(* Logix 5000 AddOnInstructionDefinition export QWX43; software revision 18.02 *)

TYPE SKT_Write_Parameters :
STRUCT
   Timeout : DINT;
   ToAddr : SKT_Address;
   Buffer : STR_480;
END_STRUCT
END_TYPE

TYPE SKT_Create_Parameters :
STRUCT
   Type : DINT;   // 1 - TCP 2- UPD
   Addr : SKT_Address;
END_STRUCT
END_TYPE

TYPE QWX43_Header :
STRUCT
   SOT : INT;   // Constant identifier that a transfer of new parameters starts. Always has the following value: 0xABCD.
   ProtocolVersion : INT;   // A version identifier of the protocol. Whenever a software version is released which has changes in the protocols (adding or removing parameters) the version is increased. The version starts with 1. Always 2
   SenderID : String40;   // PLC sends data to QWX43: OrderNr_SerialNr (null terminated string, 36 bytes long) Note: The sizes of the Sender ID is different when sending or receiving
   NrOfPar : INT;   // The total amount of transmitted parameters per transfer.
   NrOfBytes : INT;   // The total amount of bytes of all transmitted parameters.
END_STRUCT
END_TYPE

TYPE SKT_OpenConnection_Parameters :
STRUCT
   Timeout : DINT;
   DestAddr : STRING;
END_STRUCT
END_TYPE

TYPE SKT_Read_Parameters :
STRUCT
   Timeout : DINT;
   BufLen : DINT;
END_STRUCT
END_TYPE

TYPE SKT_Address :
STRUCT
   Family : INT;   // Address Family Must be 2
   Port : INT;   // Port Number
   Addr : SINT[4];   // IP Address
END_STRUCT
END_TYPE

TYPE QWX43_SensorData :
STRUCT
   temperature : REAL;   // °C
   speedOfSound : REAL;   // m/s
   viscosity : REAL;   // mPa/s
   concentrationCo2 : REAL;   // %mass
   TSOriginalGravity : REAL;   // %mass
   TSRealExtract : REAL;   // %mass
   originalGravity : REAL;   // °P
   realExtract : REAL;   // °P
   alcoholPercentMass : REAL;   // %mass
   alcoholPercentVolume : REAL;   // %vol
   densityAt20Degrees : REAL;   // g/cm³
   densityAt15Degrees : REAL;   // g/cm³
   realFermentationDegree : REAL;   // %
   fermentableSugars : REAL;   // %mass
   nonFermentableSugars : REAL;   // %mass
   apparentExtract : REAL;   // °P
   residualExtractBalling : REAL;   // °P
   alcoholBalling : REAL;   // %vol
   apparFermentationDeg : REAL;   // %
   fermentationSpeed : REAL;   // %vol/h
   viscosityAt20Degrees : REAL;   // mPa/s
   originalGravityMebak : REAL;   // °P
   realExtractMebak : REAL;   // °P
   alcoholPercentMassMebak : REAL;   // %mass
   alcoholPercentVolMebak : REAL;   // %vol
   densityAt20DegreesMebak : REAL;   // g/cm³
   densityAt15DegreesMebak : REAL;   // g/cm³
   realFermentationDegMebak : REAL;   // %
   apparentExtractMebak : REAL;   // °P
   residExtractBallingMebak : REAL;   // °P
   alcoholBallingMebak : REAL;   // %vol
   apparFermentationDegMebak : REAL;   // %
   errorCode : INT[10];   // -
   service_Temperature1 : REAL;   // °C
   service_Temperature2 : REAL;   // °C
   service_SSpeed : REAL;   // m/s
   service_SSpeedH2O : REAL;   // m/s
   service_dSSpeed : REAL;   // m/s
   service_Density45 : REAL;   // g/cm³
   service_Density : REAL;   // g/cm³
   service_DensityH2O : REAL;   // g/cm³
   service_RelDensity : REAL;   // g/cm³
   service_Viscosity : REAL;   // mPa/s
   service_TempElectronic : REAL;   // °C
   service_TOfRaw : REAL;   // s
   service_TransFrqc : REAL;   // Hz
   service_TDCError : INT;   // -
   service_DIVOFrqc : REAL;   // Hz
   service_DIVODamping : REAL;   // -
   service_DIVOCapacity : REAL;   // -
   service_DIVOStatus : REAL;   // -
   service_Uncovered : INT;   // -
END_STRUCT
END_TYPE

TYPE STR_480 :   // string type
STRUCT
   LEN : DINT;
   DATA : SINT[480];
END_STRUCT
END_TYPE

TYPE String40 :   // string type
STRUCT
   LEN : DINT;
   DATA : SINT[40];
END_STRUCT
END_TYPE

TYPE SKT_Read_Response :
STRUCT
   FromAddr : SKT_Address;
   Buffer : STR_480;
END_STRUCT
END_TYPE

TYPE SKT_DATA_CLIENT :
STRUCT
   Timeout : DINT;
   Create_Source : SKT_Create_Parameters;
   Instance : DINT;
   Connect_Source : SKT_OpenConnection_Parameters;
   Read_Source : SKT_Read_Parameters;
   Read_Response : SKT_Read_Response;
   Write_Source : SKT_Write_Parameters;
   Write_SizeSent : DINT;
END_STRUCT
END_TYPE

ADD_ON_INSTRUCTION SKT_AOI_TCP_CLIENT   (* revision 1.0, ExecutePrescan *)
VAR_IN_OUT
   Client_Data : SKT_DATA_CLIENT; {required}   // This tags holds all the data used by the messages
END_VAR
VAR_INPUT
   Enable_Socket : BOOL; {visible}   // Set by user to enable or disable socket
   Stop_On_Error : BOOL; {visible}   // If any message errors, then delete socket and stop
END_VAR
VAR_IN_OUT
   Create_MSG : MESSAGE; {required}   // Create socket
   Connect_MSG : MESSAGE; {required}   // Connect socket to server.
   Read_MSG : MESSAGE; {required}   // Message to tell socket to return any data it has recieved
   Write_MSG : MESSAGE; {required}   // Write socket message
   Delete_MSG : MESSAGE; {required}   // Delete socket
END_VAR
VAR_OUTPUT
   ENABLED : BOOL; {access Read Only, visible}   // Socket not currently open
   CONNECTING : BOOL; {access Read Only, visible}   // Trying to connect to Server.
   OPEN : BOOL; {access Read Only, visible}   // Socket connection Open
   READ : BOOL; {access Read Only, visible}   // New Data Ready - Set by AOI when a string is received, cleared by user to acknowledge
   WRITE : BOOL; {access Read Only, visible}   // Set this bit to Write Data
   ERROR : BOOL; {access Read Only, visible}   // A message had an Error
END_VAR
VAR
   State : DINT := 60;   // Current state
   lastport : DINT; {access None}
END_VAR

ROUTINE Logic   (* ladder *)
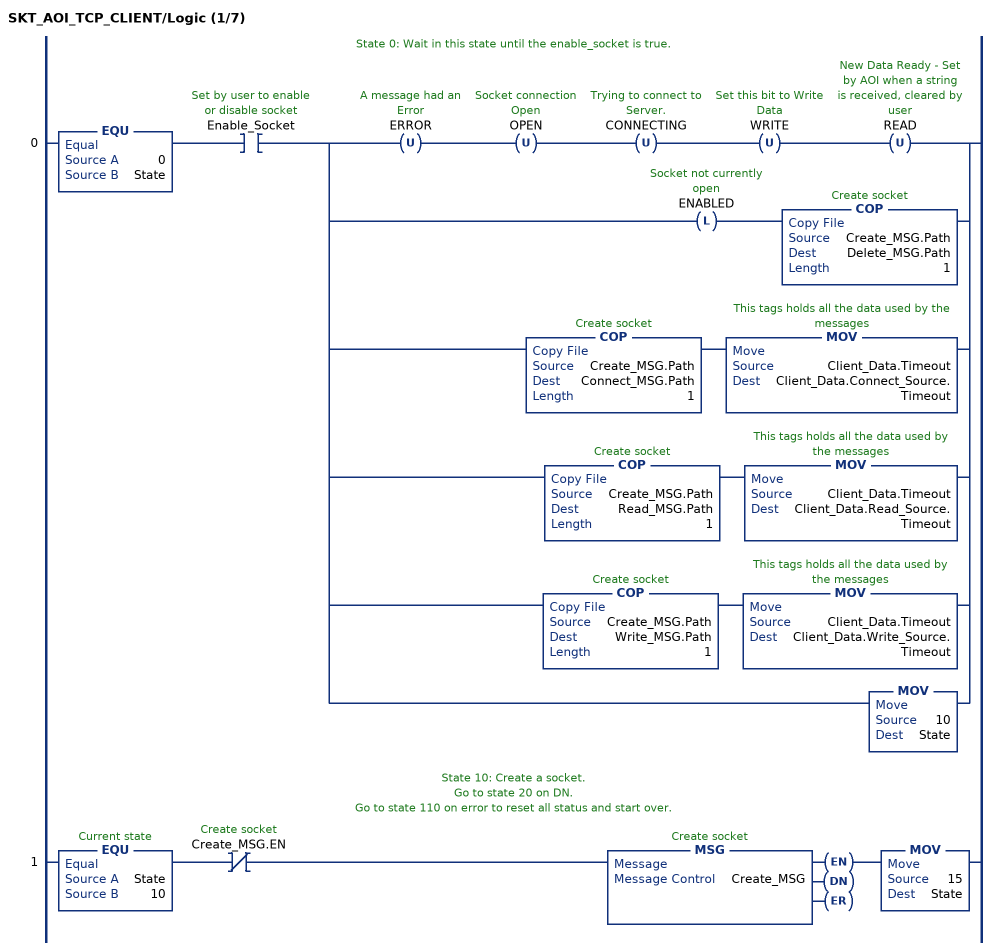
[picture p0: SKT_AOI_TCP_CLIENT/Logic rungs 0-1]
   // State 0: Wait in this state until the enable_socket is true.
   0: EQU(0,State)XIC(Enable_Socket)[OTU(ERROR) OTU(OPEN) OTU(CONNECTING) OTU(WRITE) OTU(READ) ,OTL(ENABLED) COP(Create_MSG.Path,Delete_MSG.Path,1) ,COP(Create_MSG.Path,Connect_MSG.Path,1) MOV(Client_Data.Timeout,Client_Data.Connect_Source.Timeout) ,COP(Create_MSG.Path,Read_MSG.Path,1) MOV(Client_Data.Timeout,Client_Data.Read_Source.Timeout) ,COP(Create_MSG.Path,Write_MSG.Path,1) MOV(Client_Data.Timeout,Client_Data.Write_Source.Timeout) ,MOV(10,State) ];
   // State 10: Create a socket.
   // Go to state 20 on DN.
   // Go to state 110 on error to reset all status and start over.
   1: EQU(State,10)XIO(Create_MSG.EN)MSG(Create_MSG)MOV(15,State);
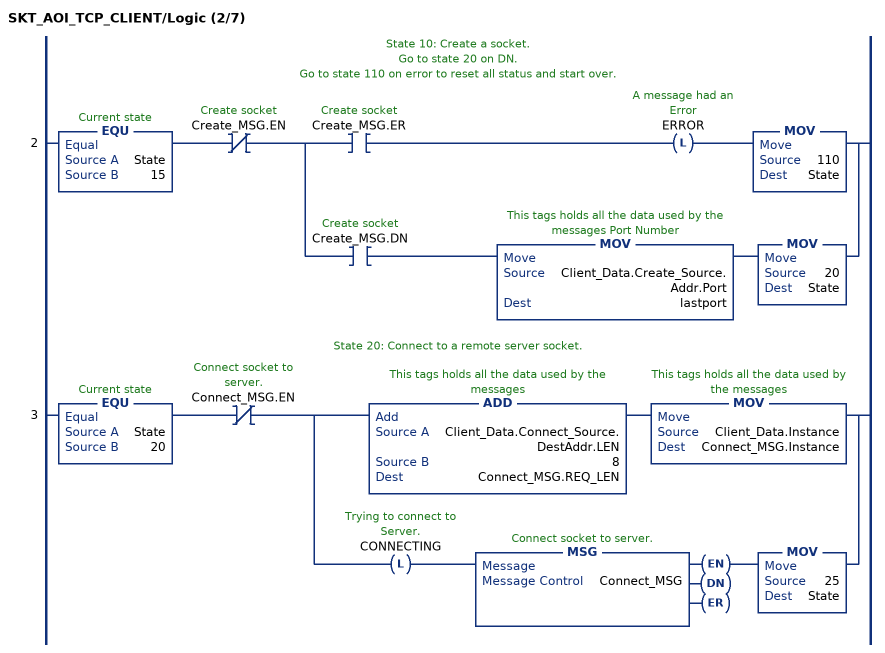
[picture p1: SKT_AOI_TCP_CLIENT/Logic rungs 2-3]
   // State 10: Create a socket.
   // Go to state 20 on DN.
   // Go to state 110 on error to reset all status and start over.
   2: EQU(State,15)XIO(Create_MSG.EN)[XIC(Create_MSG.ER) OTL(ERROR) MOV(110,State) ,XIC(Create_MSG.DN) MOV(Client_Data.Create_Source.Addr.Port,lastport) MOV(20,State) ];
   // State 20: Connect to a remote server socket.
   3: EQU(State,20)XIO(Connect_MSG.EN)[ADD(Client_Data.Connect_Source.DestAddr.LEN,8,Connect_MSG.REQ_LEN) MOV(Client_Data.Instance,Connect_MSG.Instance) ,OTL(CONNECTING) MSG(Connect_MSG) MOV(25,State) ];
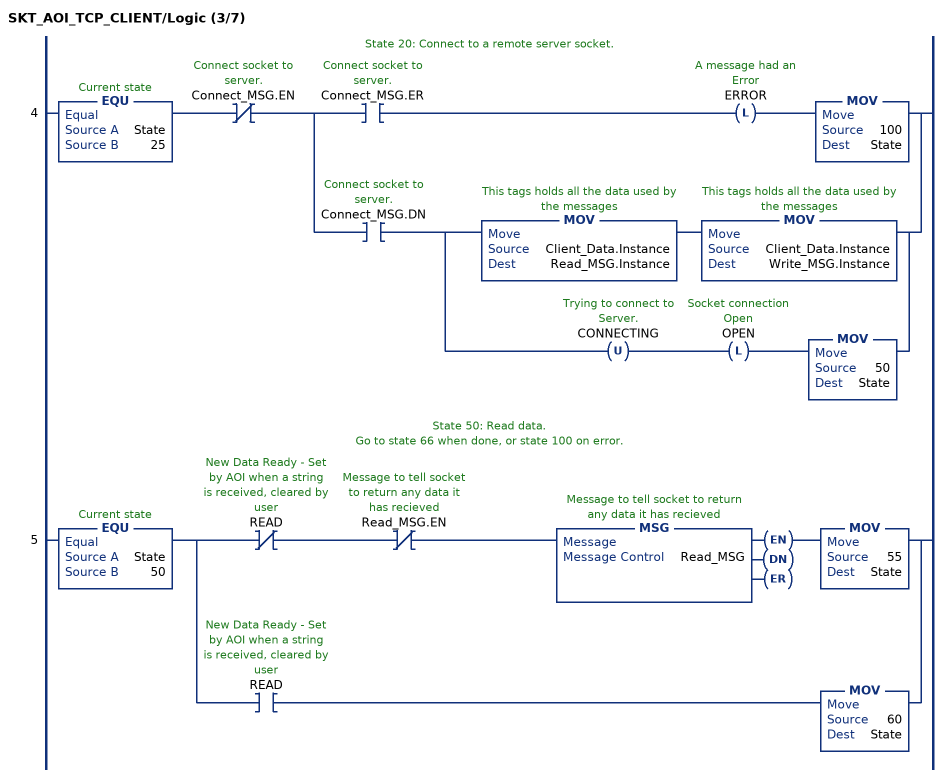
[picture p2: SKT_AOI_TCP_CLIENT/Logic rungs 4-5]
   // State 20: Connect to a remote server socket.
   4: EQU(State,25)XIO(Connect_MSG.EN)[XIC(Connect_MSG.ER) OTL(ERROR) MOV(100,State) ,XIC(Connect_MSG.DN) [MOV(Client_Data.Instance,Read_MSG.Instance) MOV(Client_Data.Instance,Write_MSG.Instance) ,OTU(CONNECTING) OTL(OPEN) MOV(50,State) ] ];
   // State 50: Read data.
   // Go to state 66 when done, or state 100 on error.
   5: EQU(State,50)[XIO(READ) XIO(Read_MSG.EN) MSG(Read_MSG) MOV(55,State) ,XIC(READ) MOV(60,State) ];
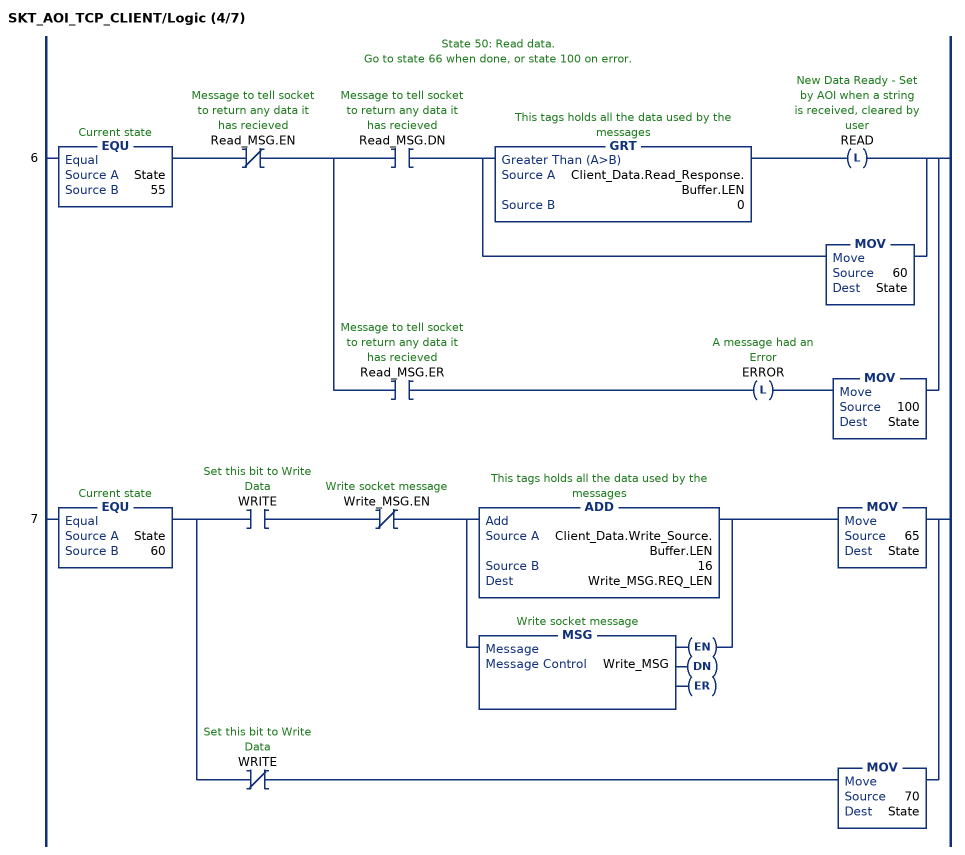
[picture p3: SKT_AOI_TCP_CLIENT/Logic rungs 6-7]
   // State 50: Read data.
   // Go to state 66 when done, or state 100 on error.
   6: EQU(State,55)XIO(Read_MSG.EN)[XIC(Read_MSG.DN) [GRT(Client_Data.Read_Response.Buffer.LEN,0) OTL(READ) ,MOV(60,State) ] ,XIC(Read_MSG.ER) OTL(ERROR) MOV(100,State) ];
   7: EQU(State,60)[XIC(WRITE) XIO(Write_MSG.EN) [ADD(Client_Data.Write_Source.Buffer.LEN,16,Write_MSG.REQ_LEN) ,MSG(Write_MSG) ] MOV(65,State) ,XIO(WRITE) MOV(70,State) ];
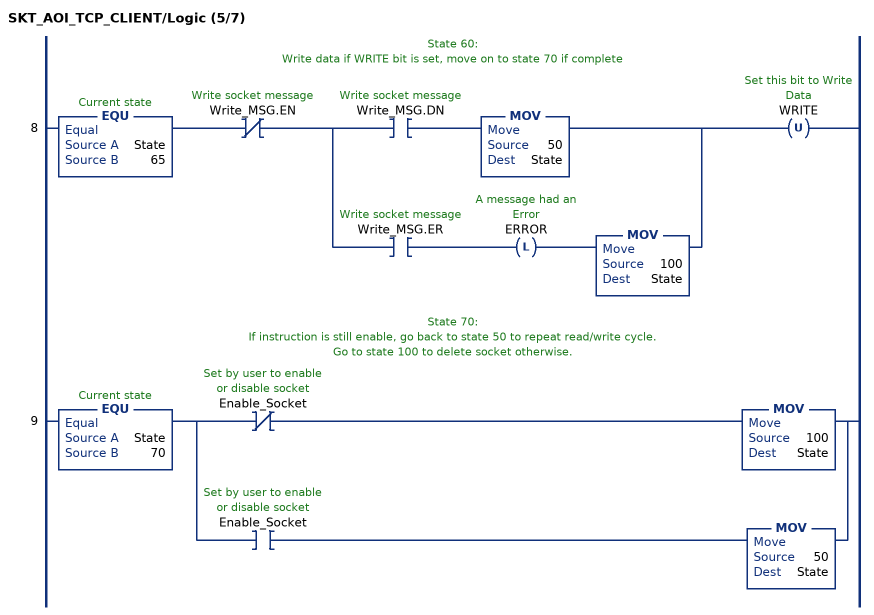
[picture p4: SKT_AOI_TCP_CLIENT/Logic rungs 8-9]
   // State 60:
   // Write data if WRITE bit is set, move on to state 70 if complete
   8: EQU(State,65)XIO(Write_MSG.EN)[XIC(Write_MSG.DN) MOV(50,State) ,XIC(Write_MSG.ER) OTL(ERROR) MOV(100,State) ]OTU(WRITE);
   // State 70:
   // If instruction is still enable, go back to state 50 to repeat read/write cycle.
   // Go to state 100 to delete socket otherwise.
   9: EQU(State,70)[XIO(Enable_Socket) MOV(100,State) ,XIC(Enable_Socket) MOV(50,State) ];
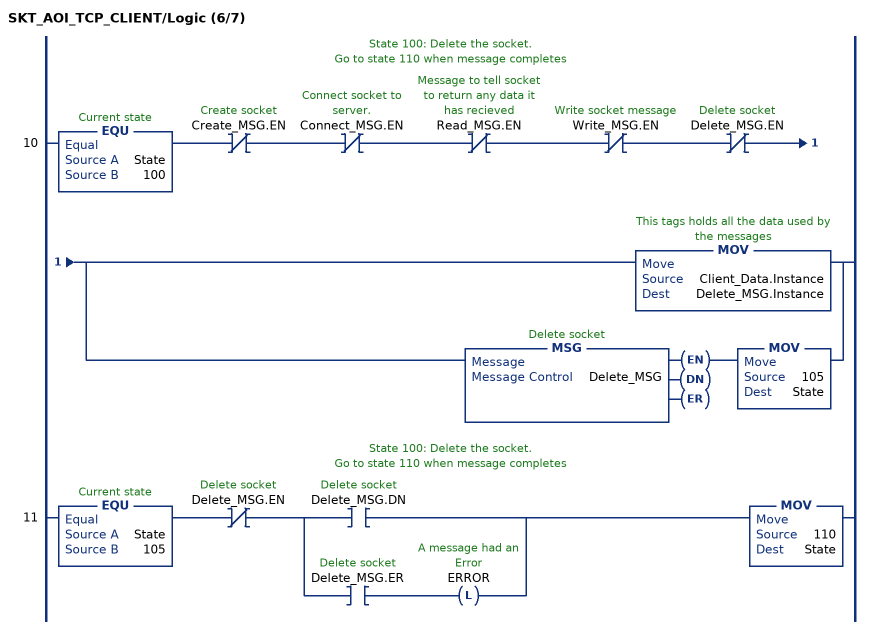
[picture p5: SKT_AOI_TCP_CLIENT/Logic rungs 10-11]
   // State 100: Delete the socket.
   // Go to state 110 when message completes
   10: EQU(State,100)XIO(Create_MSG.EN)XIO(Connect_MSG.EN)XIO(Read_MSG.EN)XIO(Write_MSG.EN)XIO(Delete_MSG.EN)[MOV(Client_Data.Instance,Delete_MSG.Instance) ,MSG(Delete_MSG) MOV(105,State) ];
   // State 100: Delete the socket.
   // Go to state 110 when message completes
   11: EQU(State,105)XIO(Delete_MSG.EN)[XIC(Delete_MSG.DN) ,XIC(Delete_MSG.ER) OTL(ERROR) ]MOV(110,State);
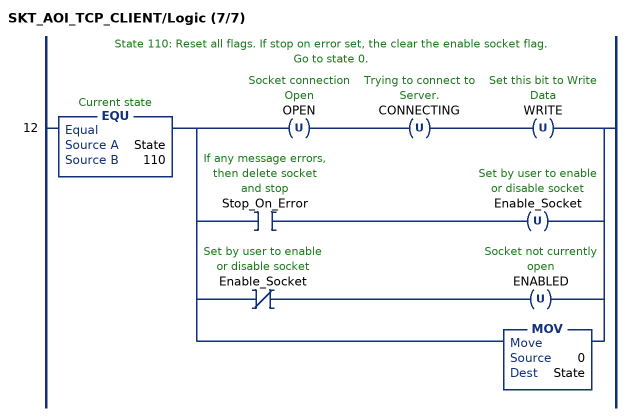
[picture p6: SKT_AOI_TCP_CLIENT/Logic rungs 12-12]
   // State 110: Reset all flags. If stop on error set, the clear the enable socket flag.
   // Go to state 0.
   12: EQU(State,110)[OTU(OPEN) OTU(CONNECTING) OTU(WRITE) ,XIC(Stop_On_Error) OTU(Enable_Socket) ,XIO(Enable_Socket) OTU(ENABLED) ,MOV(0,State) ];
END_ROUTINE

ROUTINE Prescan   (* ladder *)
// Prescan
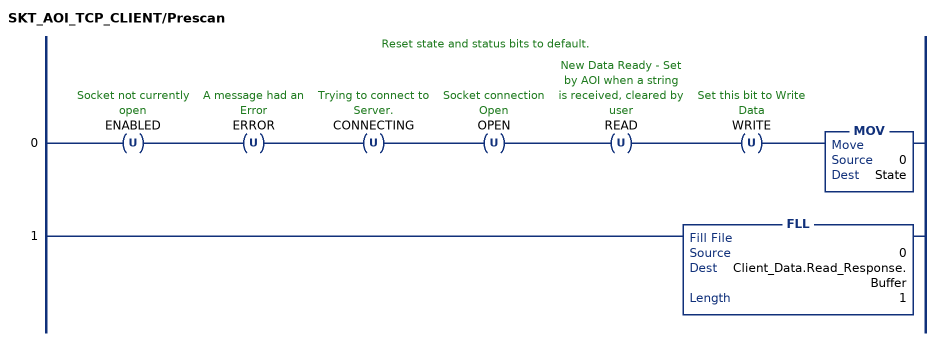
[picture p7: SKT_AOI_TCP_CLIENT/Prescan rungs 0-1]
   // Reset state and status bits to default.
   0: OTU(ENABLED)OTU(ERROR)OTU(CONNECTING)OTU(OPEN)OTU(READ)OTU(WRITE)MOV(0,State);
   1: FLL(0,Client_Data.Read_Response.Buffer,1);
END_ROUTINE
END_ADD_ON_INSTRUCTION

ADD_ON_INSTRUCTION QWX43   (* revision 1.1, vendor Endress+Hauser *)
// TCP/IP Communication to a QWX43 sensor
// Revision note:
// V1.01
// fixed that the Output Buffer was not copied to the send data
// Protocol Revision 3
// Help:
// Communication Handler for Endress+Hauser QWX43 Sensor.
// Communication is handled over TCP/IP. The Sensor will transmit and receive data on Port 50000.
// Protocol definition - Version 3
// Header [38 Bytes] - StartOfTransfer | Version | SenderID | NumberOfParameters | NrOfBytes
// Sensor Data [220 Bytes]
// Trailer [2 Bytes] - EndOfTransfer
// Revision:
// v1.0 - Initial release
// ***************************************************************************
// Message Paths
//     5570 and 5560 controllers
//         It will be 1,[Slot of ethernet module] if typed manually, or '$01$xx'if loaded programmatically to the .PATH field where xx is the HEX equivalent of decimal value of the slot. (ex. Slot 12 in HEX would be 0C)
//     5370 controllers
//         It will be 1,0 if typed manually, or '$01$00' if loaded programmatically to the .PATH field.
//     5380 controllers
//         Linear/ DLR mode
//             1,0 is the preferred recommended path to self, or '$01$00' if loaded programmatically the .PATH field.
//         Dual IP mode
//             If the controller is in dual IP mode the message path will be the same as above however the source of the CREATE MESSAGE needs to have the IP of the port that the socket will communicate
//             Reference QA48896 - 5380 Ethernet Socket Errors and Path Information  to specify the correct port the message should sent out for dual IP
// Note: 'THIS' will not work as the path for the 5380 controllers because of the dual IP capabilities use the path provided above
//     5580 controllers
//         When doing a message to self the message path should either be '1,<slot of controller>' or THIS. THIS is the preferred recommended path to self, or '$1F$00$00$00';if loaded programmatically the .PATH field.
// see also: IN37624 Socket Communication in ControlLogix, CompactLogix and MicroLogix Controllers
// https://rockwellautomation.custhelp.com/app/answers/answer_view/a_id/470690
// ***************************************************************************
// The DestAddr holds the IP and port adress of the QWX43 in the Format "192.168.1.127?port=50000"
VAR_INPUT
   Inp_Release : BOOL; {visible}   // 1= Enable communication to QWX43
   Inp_MaxPressure : REAL; {visible}   // Maximum head pressure of the tank in bar (absolute pressure)
END_VAR
VAR_IN_OUT
   SKT_DATA_Client : SKT_DATA_CLIENT; {required}   // This tags holds all the data used by the messages
   SKT_MSG_Client_Create : MESSAGE; {required}   // Create socket
   SKT_MSG_Client_Connect : MESSAGE; {required}   // Connect socket to server.
   SKT_MSG_Client_Read : MESSAGE; {required}   // Message to tell socket to return any data it has recieved
   SKT_MSG_Client_Write : MESSAGE; {required}   // Write socket message
   SKT_MSG_Client_Delete : MESSAGE; {required}   // Delete socket
   SKT_MSG_Delete_All : MESSAGE; {required}   // Delete all sockets in modul
   Out_SensorData : QWX43_SensorData; {required}   // Received Sensor Data
END_VAR
VAR_INPUT
   Cfg_ComModuleSingleUse : BOOL; {visible}   // The configured communication module is 1=only used for this QWX43 0=also used by others (default)
END_VAR
VAR_OUTPUT
   Sts_Error : BOOL; {access Read Only, visible}   // 1= functionblock is in an error state
   Sts_State : DINT; {access Read Only, visible}   // State of the function 0=Wait, 1=Connect, 2=Send, 3=Receive 100=ConfigError, 101=ConnectionError, 102=TelegramError, 103=VersionError
END_VAR
VAR
   Err_Config : BOOL; {access None}   // Error in basic configuration
   Wrk_State : DINT; {access None}   // State of the function 0=Wait, 1=Connect, 2=Send, 3=Receive 100=ConfigError, 101=ConnectionError, 102=TelegramError, 103=VersionError
   ons : DINT; {access None}
   Wrk_Connected : BOOL; {access None}   // Socket is connected to the QWX43
   SKT_AOI_Client : SKT_AOI_TCP_CLIENT;   // Socket handling
   Wrk_SendInterval_T : TIMER := (PRE := 1000); {access None}
   cSOT : INT := 16#abcd; {access None}   // 0xABCD
   cEOT : INT := 16#fedc; {access None}   // 0xFEDC
   Wrk_SendHeader : QWX43_Header := (SOT := 16#abcd, ProtocolVersion := 3, SenderID := 'CLX', NrOfPar := 2, NrOfBytes := 6); {access None}
   Wrk_ReceiveHeader : QWX43_Header; {access None}
   Wrk_SendBytes : DINT := 56; {access None}
   Cfg_BytesHeader : DINT := 48; {access None}   // Number of bytes in header
   Cfg_BytesTrailer : DINT := 2; {access None}   // Number of bytes in trailer
   Cfg_BytesSendData : DINT := 6; {access None}   // Number of bytes in send data
   Wrk_SendBuffer : STR_480; {access None}
   Wrk_SendByteOffset : DINT; {access None}
   Wrk_SendByteLen : DINT; {access None}
   Wrk_dummyINT : INT; {access None}
   Wrk_ErrorCodePLC : INT; {access None}   // 0=no error (not used at the moment)
   Wrk_dummyDINT : DINT; {access None}
   Wrk_ReceiveBuffer : STR_480; {access None}
   Err_ReceiveDataLenNOK : BOOL; {access None}   // The received data lengh did not match
   Err_ReceiveHeaderDataNOK : BOOL; {access None}   // At least one of the received header data was incorrect
   Wrk_ReceiveBytesExpected : DINT := 270; {access None}   // Expected number of bytes to receive
   Cfg_BytesReceiveData : DINT := 220; {access None}   // Number of bytes in receive data
   Wrk_ReceiveByteOffset : DINT; {access None}
   Wrk_ReceiveByteLen : DINT; {access None}
   Wrk_ReceiveByteOffsetEOT : DINT; {access None}
   Wrk_ReceiveEOT : INT; {access None}
   Wrk_ReceiveSwapIndex : DINT; {access None}
   Wrk_ReceiveSwapNo : DINT; {access None}   // Number of data elements to swap
   Wrk_ReceiveSwapSize : DINT; {access None}   // Number of bytes per element to swap
   Wrk_dummyDINT_A : DINT[100]; {access None}
   Wrk_dummyINT_A : INT[100]; {access None}
   Wrk_dummyDINT_A_Size : DINT; {access None}
   Wrk_dummyINT_A_Size : DINT; {access None}
   Wrk_ReceiveBuffer_Size : DINT := 480; {access None}
   Wrk_SendBuffer_Size : DINT := 480; {access None}
   Err_ReceiveVersionNOK : BOOL; {access None}   // The received data version is incorrect
   Err_Connection : BOOL; {access None}   // No connection could be established
   Wrk_ConnectingError_T : TIMER := (PRE := 5000); {access None}
   Err_ConnectionTimeout : BOOL; {access None}   // Timeout after a connection was established
   Wrk_ConnectionTimeout_T : TIMER := (PRE := 5000); {access None}
   Wrk_CloseSocket : BOOL; {access None}   // Temporary close socket after a timeout
   Wrk_ConnectionTimeoutWait_T : TIMER := (PRE := 15000); {access None}
   Cfg_ConnectionTimeout : DINT := 5000; {access None}   // Timeout after a connection was opened, no data received [ms]
   Cfg_ConnectionTimeoutWait : DINT := 15000; {access None}   // Wait after a timeout befor trying to reconnect [ms]
   Cfg_ConnectionError : DINT := 5000; {access None}   // A connection could not be established [ms]
   Cfg_SendInterval : DINT := 1000; {access None}   // Intervaltime [ms]
   Err_MSGDeleteAll : BOOL; {access None}   // The MSG Delete All had an error
END_VAR

ROUTINE Logic   (* ladder *)
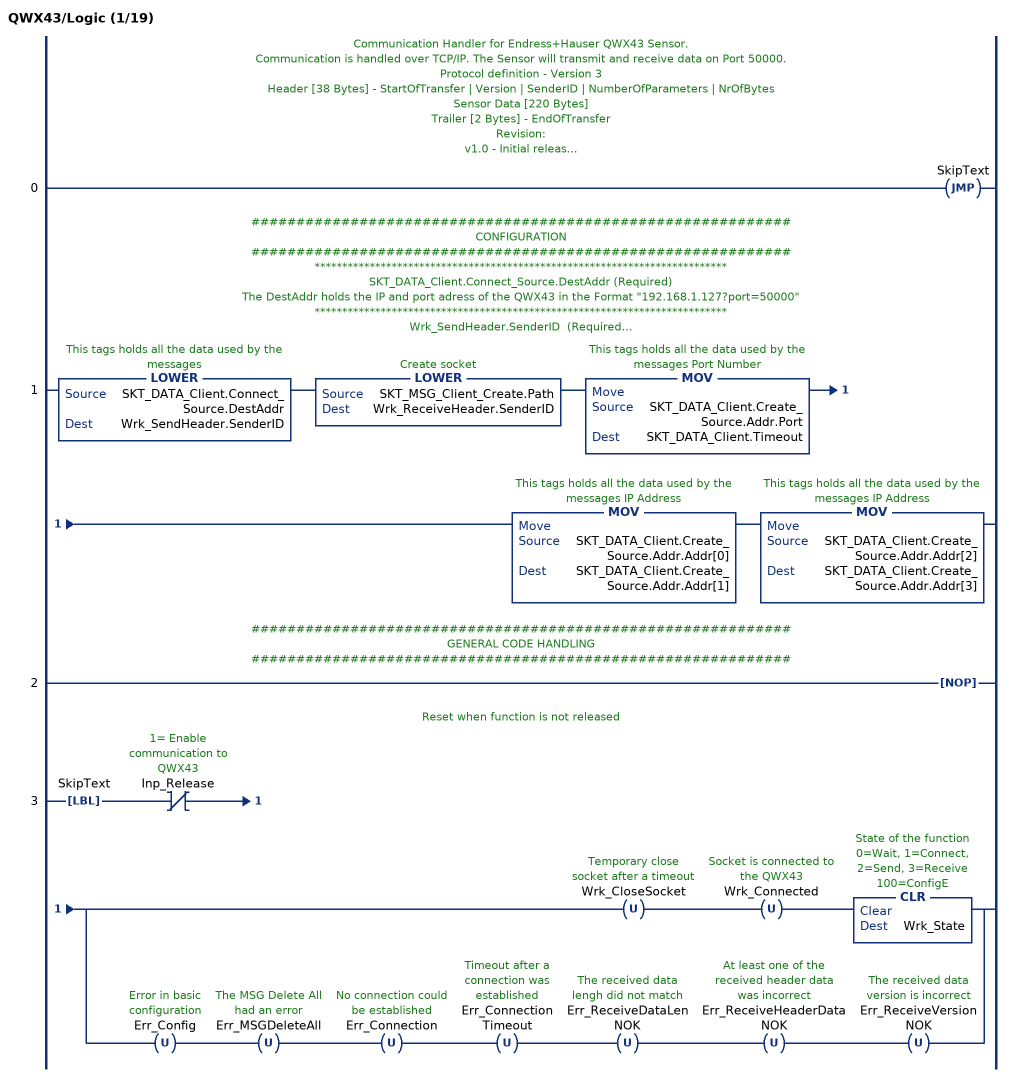
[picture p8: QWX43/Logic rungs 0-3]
   // Communication Handler for Endress+Hauser QWX43 Sensor.
   // Communication is handled over TCP/IP. The Sensor will transmit and receive data on Port 50000.
   // Protocol definition - Version 3
   // Header [38 Bytes] - StartOfTransfer | Version | SenderID | NumberOfParameters | NrOfBytes
   // Sensor Data [220 Bytes]
   // Trailer [2 Bytes] - EndOfTransfer
   // Revision:
   // v1.0 - Initial release
   // ***************************************************************************
   // In order to make it easier to find and configure these STRINGs, this rung
   // was added.  THE JMP (and the LBL on the following rung)
   // MUST NOT BE REMOVED!!!
   0: JMP(SkipText);
   // ############################################################
   // CONFIGURATION
   // ############################################################
   // ***************************************************************************
   // SKT_DATA_Client.Connect_Source.DestAddr (Required)
   // The DestAddr holds the IP and port adress of the QWX43 in the Format "192.168.1.127?port=50000"
   // ***************************************************************************
   // Wrk_SendHeader.SenderID  (Required)
   // This is a String which holds the Sender ID of the PLC (max 36 characters)
   // ***************************************************************************
   // SKT_MSG_Client_Create.Path  (Required, either here manualy or at the MSG instance at the AOI)
   // Message Paths
   //     5570 and 5560 controllers
   //         It will be 1,[Slot of ethernet module] if typed manually, or '$01$xx'if loaded programmatically to the .PATH field where xx is the HEX equivalent of decimal value of the slot. (ex. Slot 12 in HEX would be 0C)
   //     5370 controllers
   //         It will be 1,0 if typed manually, or '$01$00' if loaded programmatically to the .PATH field.
   //     5380 controllers
   //         Linear/ DLR mode
   //             1,0 is the preferred recommended path to self, or '$01$00' if loaded programmatically the .PATH field.
   //         Dual IP mode
   //             If the controller is in dual IP mode the message path will be the same as above however the source of the CREATE MESSAGE needs to have the IP of the port that the socket will communicate
   //             Reference QA48896 - 5380 Ethernet Socket Errors and Path Information  to specify the correct port the message should sent out for dual IP
   // Note: 'THIS' will not work as the path for the 5380 controllers because of the dual IP capabilities use the path provided above
   //     5580 controllers
   //         When doing a message to self the message path should either be '1,<slot of controller>' or THIS. THIS is the preferred recommended path to self, or '$1F$00$00$00';if loaded programmatically the .PATH field.
   // see also: IN37624 Socket Communication in ControlLogix, CompactLogix and MicroLogix Controllers
   // https://rockwellautomation.custhelp.com/app/answers/answer_view/a_id/470690
   // ***************************************************************************
   // Wrk_ReceiveHeader.SenderID (Only to visualize)
   // The Sender ID received from the QWX43
   // ***************************************************************************
   // SKT_DATA_Client.Create_Source.Addr.Port (Otpional)
   // Specify the local port number on which an application listens and receives. (Values 1 - 32767)
   // If you want a port that is randomly assigned, use port 0 (Default).
   // ***************************************************************************
   // SKT_DATA_Client.Timeout (Optional)
   // Defines how long the read instruction will wait for new data and block a write command
   // slower values is better for response time after a write command but increases the burden on th ecommunication module
   // the default value of 100ms should fit in most cases.
   // ***************************************************************************
   // SKT_DATA_Client.Create_Source.Addr.Addr[0] - [3] (Required for Dual IP)
   // When dual IP is used (for example with Compact Logix CPUs) then the IP address of the used Port must be configured.
   // Addr[0] holds the first (lowest) octet and Addr[3] thie last (highest) octet in HEX
   // for example: 192.168.1.11 would be:
   // Addr[0] = 16#0b (11)
   // Addr[1] = 16#01 (1)
   // Addr[2] = 16#a8 (168)
   // Addr[3] = 16#c0 (192)
   // If this function is not used then all four values have to be 0 !!!
   1: LOWER(SKT_DATA_Client.Connect_Source.DestAddr,Wrk_SendHeader.SenderID)LOWER(SKT_MSG_Client_Create.Path,Wrk_ReceiveHeader.SenderID)MOV(SKT_DATA_Client.Create_Source.Addr.Port,SKT_DATA_Client.Timeout)MOV(SKT_DATA_Client.Create_Source.Addr.Addr[0],SKT_DATA_Client.Create_Source.Addr.Addr[1])MOV(SKT_DATA_Client.Create_Source.Addr.Addr[2],SKT_DATA_Client.Create_Source.Addr.Addr[3]);
   // ############################################################
   // GENERAL CODE HANDLING
   // ############################################################
   2: NOP();
   // Reset when function is not released
   3: LBL(SkipText)XIO(Inp_Release)[OTU(Wrk_CloseSocket) OTU(Wrk_Connected) CLR(Wrk_State) ,OTU(Err_Config) OTU(Err_MSGDeleteAll) OTU(Err_Connection) OTU(Err_ConnectionTimeout) OTU(Err_ReceiveDataLenNOK) OTU(Err_ReceiveHeaderDataNOK) OTU(Err_ReceiveVersionNOK) ];
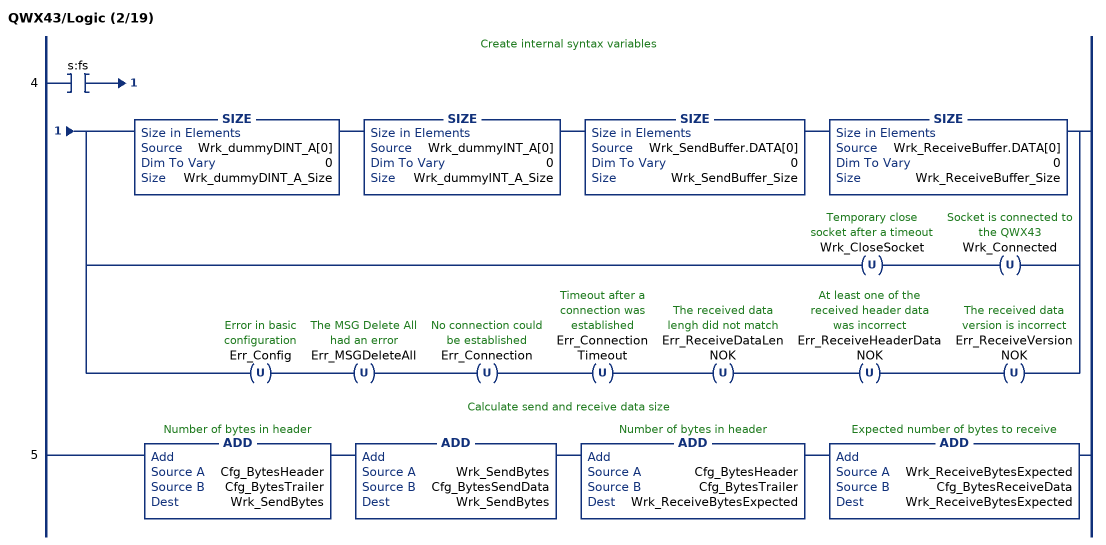
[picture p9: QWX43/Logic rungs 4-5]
   // Create internal syntax variables
   4: XIC(s:fs)[SIZE(Wrk_dummyDINT_A[0],0,Wrk_dummyDINT_A_Size) SIZE(Wrk_dummyINT_A[0],0,Wrk_dummyINT_A_Size) SIZE(Wrk_SendBuffer.DATA[0],0,Wrk_SendBuffer_Size) SIZE(Wrk_ReceiveBuffer.DATA[0],0,Wrk_ReceiveBuffer_Size) ,OTU(Wrk_CloseSocket) OTU(Wrk_Connected) ,OTU(Err_Config) OTU(Err_MSGDeleteAll) OTU(Err_Connection) OTU(Err_ConnectionTimeout) OTU(Err_ReceiveDataLenNOK) OTU(Err_ReceiveHeaderDataNOK) OTU(Err_ReceiveVersionNOK) ];
   // Calculate send and receive data size
   5: ADD(Cfg_BytesHeader,Cfg_BytesTrailer,Wrk_SendBytes)ADD(Wrk_SendBytes,Cfg_BytesSendData,Wrk_SendBytes)ADD(Cfg_BytesHeader,Cfg_BytesTrailer,Wrk_ReceiveBytesExpected)ADD(Wrk_ReceiveBytesExpected,Cfg_BytesReceiveData,Wrk_ReceiveBytesExpected);
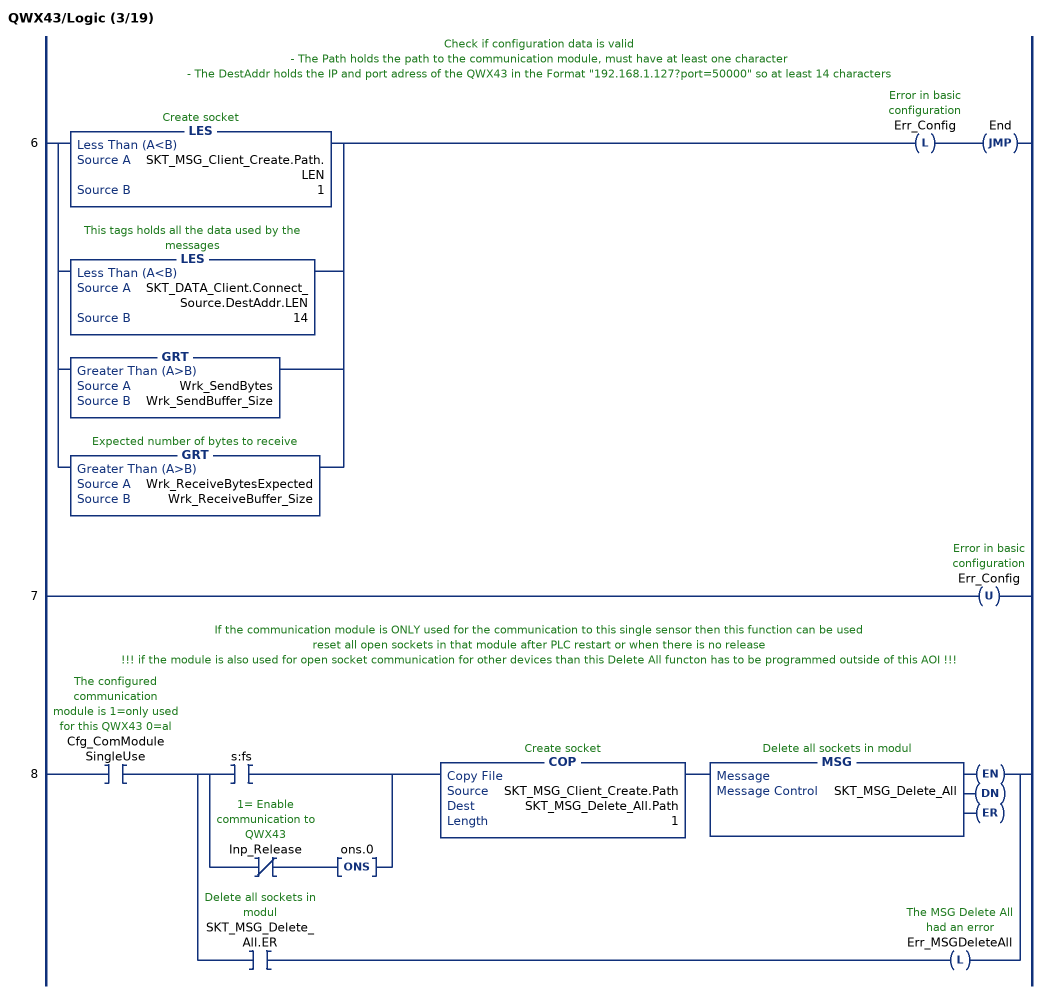
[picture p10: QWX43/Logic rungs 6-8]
   // Check if configuration data is valid
   // - The Path holds the path to the communication module, must have at least one character
   // - The DestAddr holds the IP and port adress of the QWX43 in the Format "192.168.1.127?port=50000" so at least 14 characters
   6: [LES(SKT_MSG_Client_Create.Path.LEN,1) ,LES(SKT_DATA_Client.Connect_Source.DestAddr.LEN,14) ,GRT(Wrk_SendBytes,Wrk_SendBuffer_Size) ,GRT(Wrk_ReceiveBytesExpected,Wrk_ReceiveBuffer_Size) ]OTL(Err_Config)JMP(End);
   7: OTU(Err_Config);
   // If the communication module is ONLY used for the communication to this single sensor then this function can be used
   // reset all open sockets in that module after PLC restart or when there is no release
   // !!! if the module is also used for open socket communication for other devices than this Delete All functon has to be programmed outside of this AOI !!!
   8: XIC(Cfg_ComModuleSingleUse)[[XIC(s:fs) ,XIO(Inp_Release) ONS(ons.0) ] COP(SKT_MSG_Client_Create.Path,SKT_MSG_Delete_All.Path,1) MSG(SKT_MSG_Delete_All) ,XIC(SKT_MSG_Delete_All.ER) OTL(Err_MSGDeleteAll) ];
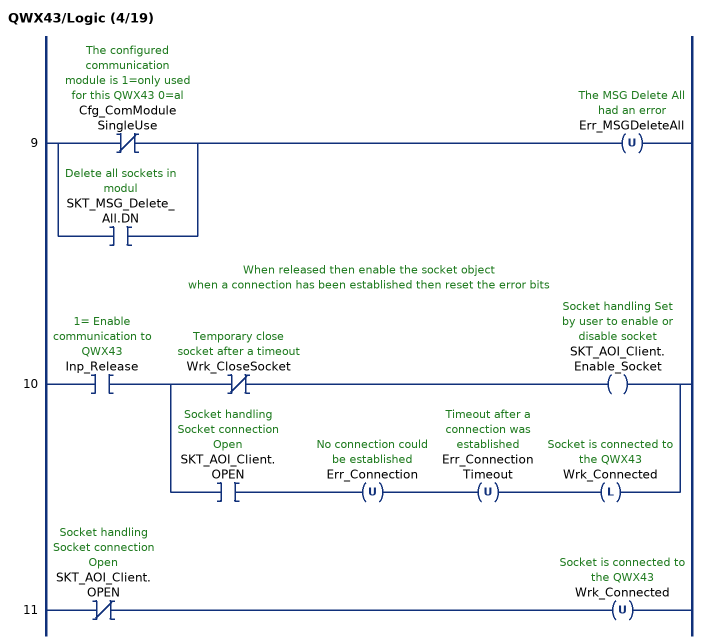
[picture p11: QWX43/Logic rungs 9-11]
   9: [XIO(Cfg_ComModuleSingleUse) ,XIC(SKT_MSG_Delete_All.DN) ]OTU(Err_MSGDeleteAll);
   // When released then enable the socket object
   // when a connection has been established then reset the error bits
   10: XIC(Inp_Release)[XIO(Wrk_CloseSocket) OTE(SKT_AOI_Client.Enable_Socket) ,XIC(SKT_AOI_Client.OPEN) OTU(Err_Connection) OTU(Err_ConnectionTimeout) OTL(Wrk_Connected) ];
   11: XIO(SKT_AOI_Client.OPEN)OTU(Wrk_Connected);
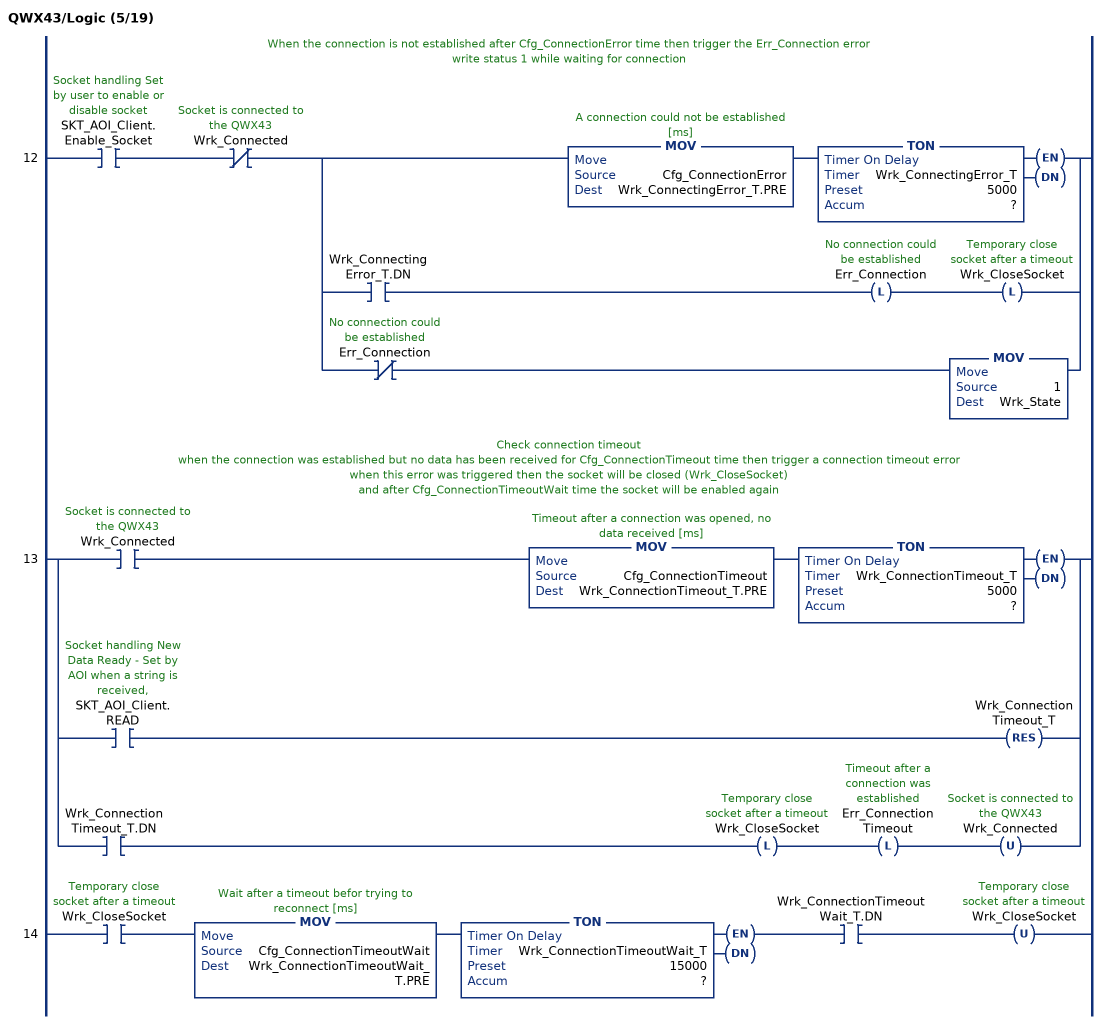
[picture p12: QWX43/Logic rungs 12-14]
   // When the connection is not established after Cfg_ConnectionError time then trigger the Err_Connection error
   // write status 1 while waiting for connection
   12: XIC(SKT_AOI_Client.Enable_Socket)XIO(Wrk_Connected)[MOV(Cfg_ConnectionError,Wrk_ConnectingError_T.PRE) TON(Wrk_ConnectingError_T,?,?) ,XIC(Wrk_ConnectingError_T.DN) OTL(Err_Connection) OTL(Wrk_CloseSocket) ,XIO(Err_Connection) MOV(1,Wrk_State) ];
   // Check connection timeout
   // when the connection was established but no data has been received for Cfg_ConnectionTimeout time then trigger a connection timeout error
   // when this error was triggered then the socket will be closed (Wrk_CloseSocket)
   // and after Cfg_ConnectionTimeoutWait time the socket will be enabled again
   13: [XIC(Wrk_Connected) MOV(Cfg_ConnectionTimeout,Wrk_ConnectionTimeout_T.PRE) TON(Wrk_ConnectionTimeout_T,?,?) ,XIC(SKT_AOI_Client.READ) RES(Wrk_ConnectionTimeout_T) ,XIC(Wrk_ConnectionTimeout_T.DN) OTL(Wrk_CloseSocket) OTL(Err_ConnectionTimeout) OTU(Wrk_Connected) ];
   14: XIC(Wrk_CloseSocket)MOV(Cfg_ConnectionTimeoutWait,Wrk_ConnectionTimeoutWait_T.PRE)TON(Wrk_ConnectionTimeoutWait_T,?,?)XIC(Wrk_ConnectionTimeoutWait_T.DN)OTU(Wrk_CloseSocket);
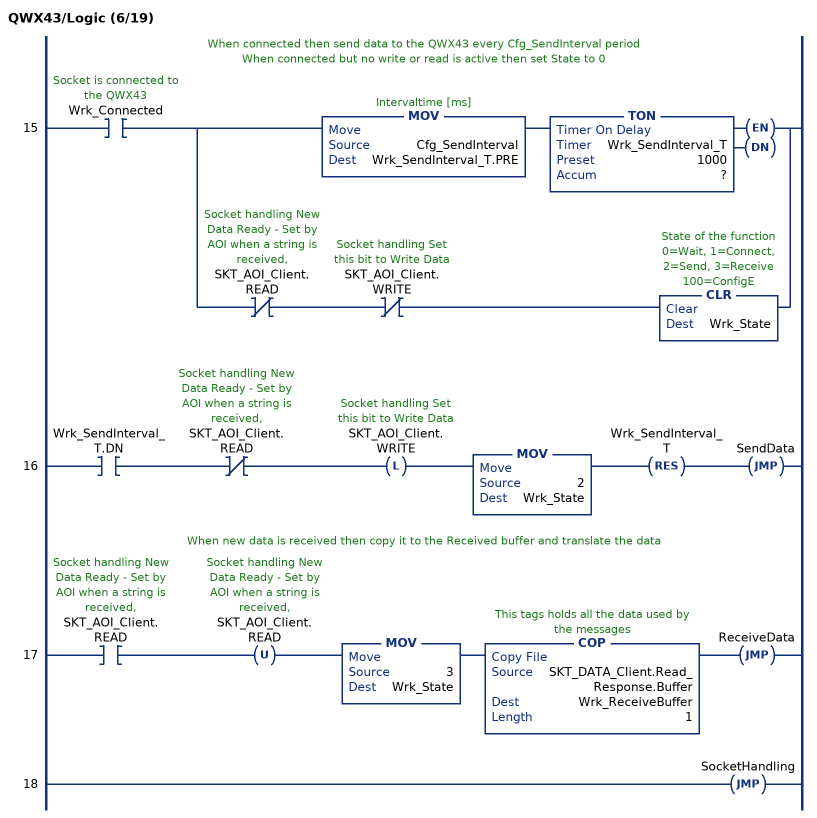
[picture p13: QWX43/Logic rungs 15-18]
   // When connected then send data to the QWX43 every Cfg_SendInterval period
   // When connected but no write or read is active then set State to 0
   15: XIC(Wrk_Connected)[MOV(Cfg_SendInterval,Wrk_SendInterval_T.PRE) TON(Wrk_SendInterval_T,?,?) ,XIO(SKT_AOI_Client.READ) XIO(SKT_AOI_Client.WRITE) CLR(Wrk_State) ];
   16: XIC(Wrk_SendInterval_T.DN)XIO(SKT_AOI_Client.READ)OTL(SKT_AOI_Client.WRITE)MOV(2,Wrk_State)RES(Wrk_SendInterval_T)JMP(SendData);
   // When new data is received then copy it to the Received buffer and translate the data
   17: XIC(SKT_AOI_Client.READ)OTU(SKT_AOI_Client.READ)MOV(3,Wrk_State)COP(SKT_DATA_Client.Read_Response.Buffer,Wrk_ReceiveBuffer,1)JMP(ReceiveData);
   18: JMP(SocketHandling);
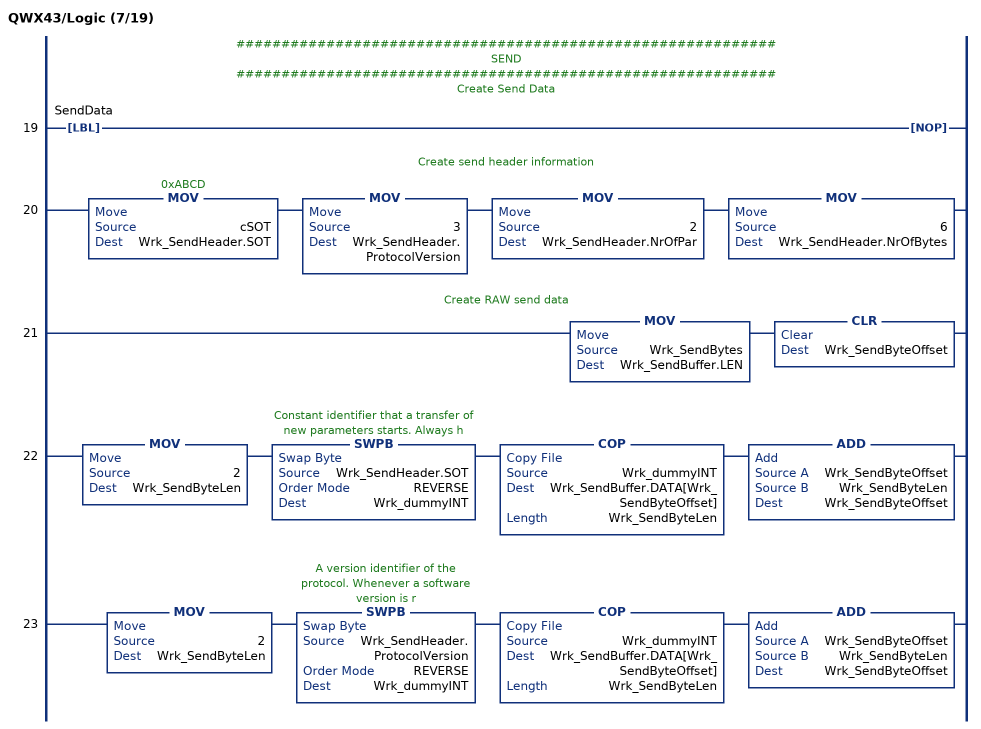
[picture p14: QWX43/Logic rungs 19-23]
   // ############################################################
   // SEND
   // ############################################################
   // Create Send Data
   19: LBL(SendData)NOP();
   // Create send header information
   20: MOV(cSOT,Wrk_SendHeader.SOT)MOV(3,Wrk_SendHeader.ProtocolVersion)MOV(2,Wrk_SendHeader.NrOfPar)MOV(6,Wrk_SendHeader.NrOfBytes);
   // Create RAW send data
   21: MOV(Wrk_SendBytes,Wrk_SendBuffer.LEN)CLR(Wrk_SendByteOffset);
   22: MOV(2,Wrk_SendByteLen)SWPB(Wrk_SendHeader.SOT,REVERSE,Wrk_dummyINT)COP(Wrk_dummyINT,Wrk_SendBuffer.DATA[Wrk_SendByteOffset],Wrk_SendByteLen)ADD(Wrk_SendByteOffset,Wrk_SendByteLen,Wrk_SendByteOffset);
   23: MOV(2,Wrk_SendByteLen)SWPB(Wrk_SendHeader.ProtocolVersion,REVERSE,Wrk_dummyINT)COP(Wrk_dummyINT,Wrk_SendBuffer.DATA[Wrk_SendByteOffset],Wrk_SendByteLen)ADD(Wrk_SendByteOffset,Wrk_SendByteLen,Wrk_SendByteOffset);
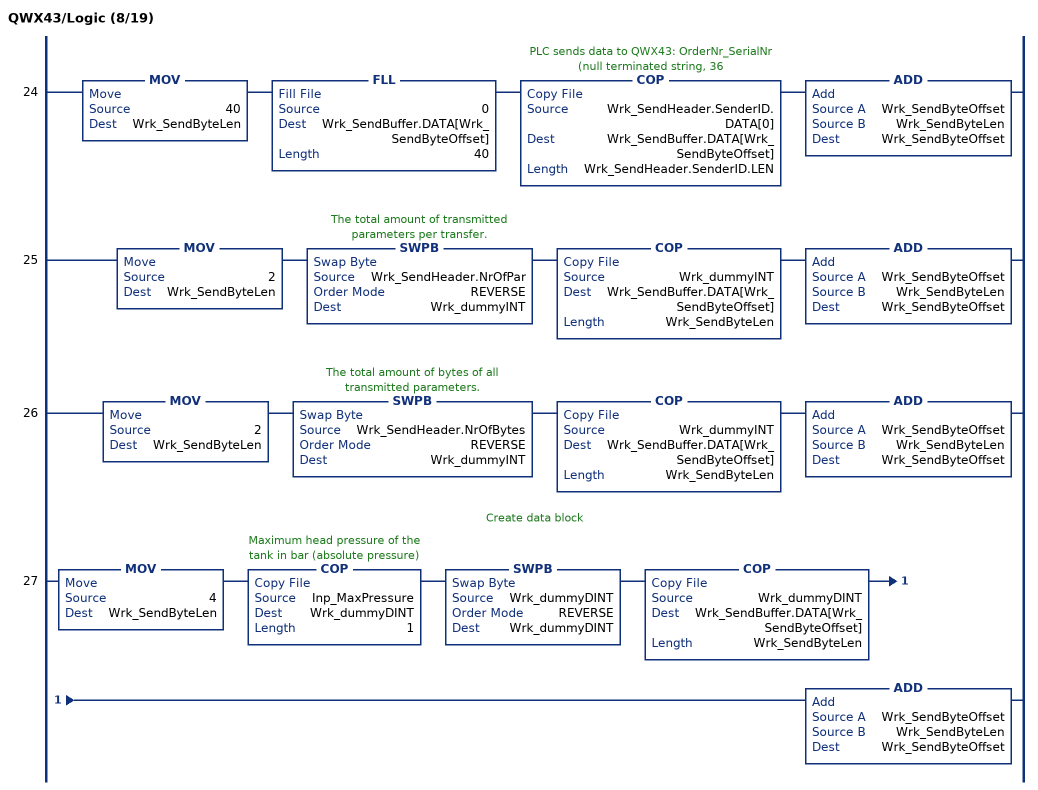
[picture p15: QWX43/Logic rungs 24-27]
   24: MOV(40,Wrk_SendByteLen)FLL(0,Wrk_SendBuffer.DATA[Wrk_SendByteOffset],40)COP(Wrk_SendHeader.SenderID.DATA[0],Wrk_SendBuffer.DATA[Wrk_SendByteOffset],Wrk_SendHeader.SenderID.LEN)ADD(Wrk_SendByteOffset,Wrk_SendByteLen,Wrk_SendByteOffset);
   25: MOV(2,Wrk_SendByteLen)SWPB(Wrk_SendHeader.NrOfPar,REVERSE,Wrk_dummyINT)COP(Wrk_dummyINT,Wrk_SendBuffer.DATA[Wrk_SendByteOffset],Wrk_SendByteLen)ADD(Wrk_SendByteOffset,Wrk_SendByteLen,Wrk_SendByteOffset);
   26: MOV(2,Wrk_SendByteLen)SWPB(Wrk_SendHeader.NrOfBytes,REVERSE,Wrk_dummyINT)COP(Wrk_dummyINT,Wrk_SendBuffer.DATA[Wrk_SendByteOffset],Wrk_SendByteLen)ADD(Wrk_SendByteOffset,Wrk_SendByteLen,Wrk_SendByteOffset);
   // Create data block
   27: MOV(4,Wrk_SendByteLen)COP(Inp_MaxPressure,Wrk_dummyDINT,1)SWPB(Wrk_dummyDINT,REVERSE,Wrk_dummyDINT)COP(Wrk_dummyDINT,Wrk_SendBuffer.DATA[Wrk_SendByteOffset],Wrk_SendByteLen)ADD(Wrk_SendByteOffset,Wrk_SendByteLen,Wrk_SendByteOffset);
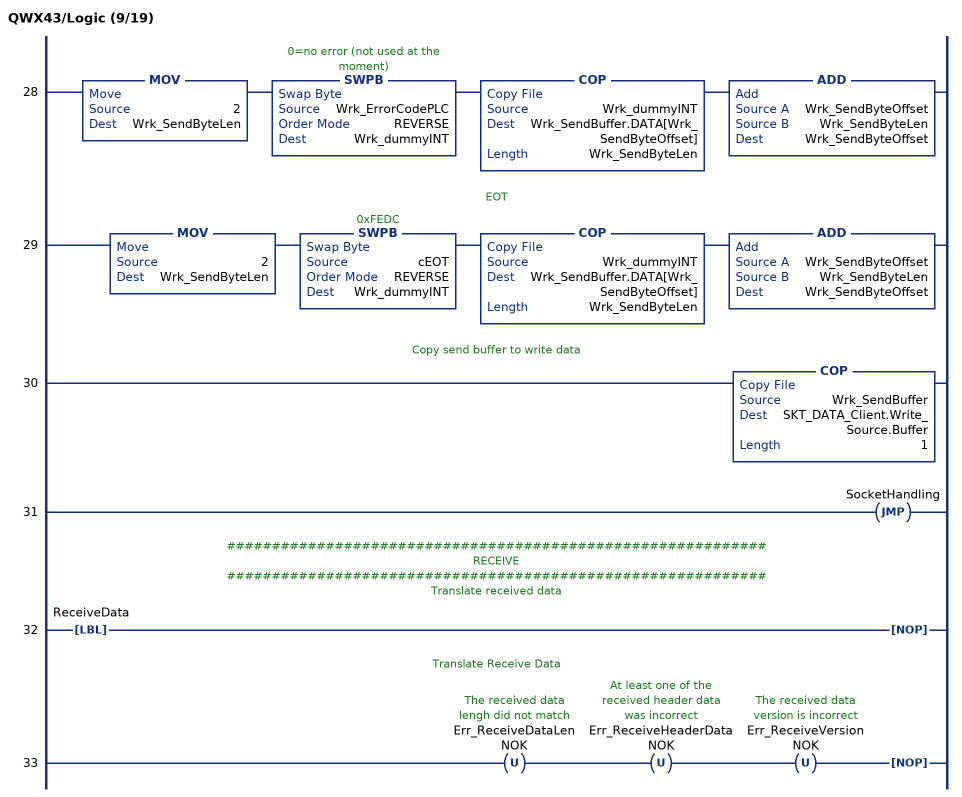
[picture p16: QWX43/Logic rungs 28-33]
   28: MOV(2,Wrk_SendByteLen)SWPB(Wrk_ErrorCodePLC,REVERSE,Wrk_dummyINT)COP(Wrk_dummyINT,Wrk_SendBuffer.DATA[Wrk_SendByteOffset],Wrk_SendByteLen)ADD(Wrk_SendByteOffset,Wrk_SendByteLen,Wrk_SendByteOffset);
   // EOT
   29: MOV(2,Wrk_SendByteLen)SWPB(cEOT,REVERSE,Wrk_dummyINT)COP(Wrk_dummyINT,Wrk_SendBuffer.DATA[Wrk_SendByteOffset],Wrk_SendByteLen)ADD(Wrk_SendByteOffset,Wrk_SendByteLen,Wrk_SendByteOffset);
   // Copy send buffer to write data
   30: COP(Wrk_SendBuffer,SKT_DATA_Client.Write_Source.Buffer,1);
   31: JMP(SocketHandling);
   // ############################################################
   // RECEIVE
   // ############################################################
   // Translate received data
   32: LBL(ReceiveData)NOP();
   // Translate Receive Data
   33: OTU(Err_ReceiveDataLenNOK)OTU(Err_ReceiveHeaderDataNOK)OTU(Err_ReceiveVersionNOK)NOP();
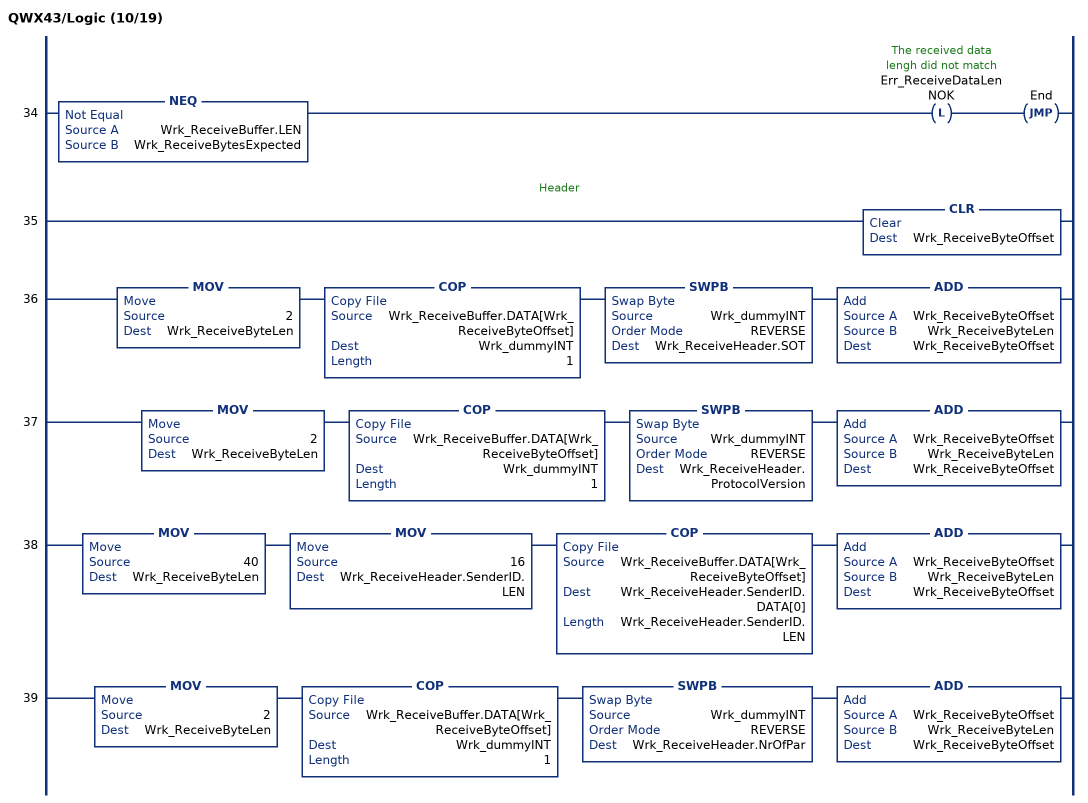
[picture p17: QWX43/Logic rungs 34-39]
   34: NEQ(Wrk_ReceiveBuffer.LEN,Wrk_ReceiveBytesExpected)OTL(Err_ReceiveDataLenNOK)JMP(End);
   // Header
   35: CLR(Wrk_ReceiveByteOffset);
   36: MOV(2,Wrk_ReceiveByteLen)COP(Wrk_ReceiveBuffer.DATA[Wrk_ReceiveByteOffset],Wrk_dummyINT,1)SWPB(Wrk_dummyINT,REVERSE,Wrk_ReceiveHeader.SOT)ADD(Wrk_ReceiveByteOffset,Wrk_ReceiveByteLen,Wrk_ReceiveByteOffset);
   37: MOV(2,Wrk_ReceiveByteLen)COP(Wrk_ReceiveBuffer.DATA[Wrk_ReceiveByteOffset],Wrk_dummyINT,1)SWPB(Wrk_dummyINT,REVERSE,Wrk_ReceiveHeader.ProtocolVersion)ADD(Wrk_ReceiveByteOffset,Wrk_ReceiveByteLen,Wrk_ReceiveByteOffset);
   38: MOV(40,Wrk_ReceiveByteLen)MOV(16,Wrk_ReceiveHeader.SenderID.LEN)COP(Wrk_ReceiveBuffer.DATA[Wrk_ReceiveByteOffset],Wrk_ReceiveHeader.SenderID.DATA[0],Wrk_ReceiveHeader.SenderID.LEN)ADD(Wrk_ReceiveByteOffset,Wrk_ReceiveByteLen,Wrk_ReceiveByteOffset);
   39: MOV(2,Wrk_ReceiveByteLen)COP(Wrk_ReceiveBuffer.DATA[Wrk_ReceiveByteOffset],Wrk_dummyINT,1)SWPB(Wrk_dummyINT,REVERSE,Wrk_ReceiveHeader.NrOfPar)ADD(Wrk_ReceiveByteOffset,Wrk_ReceiveByteLen,Wrk_ReceiveByteOffset);
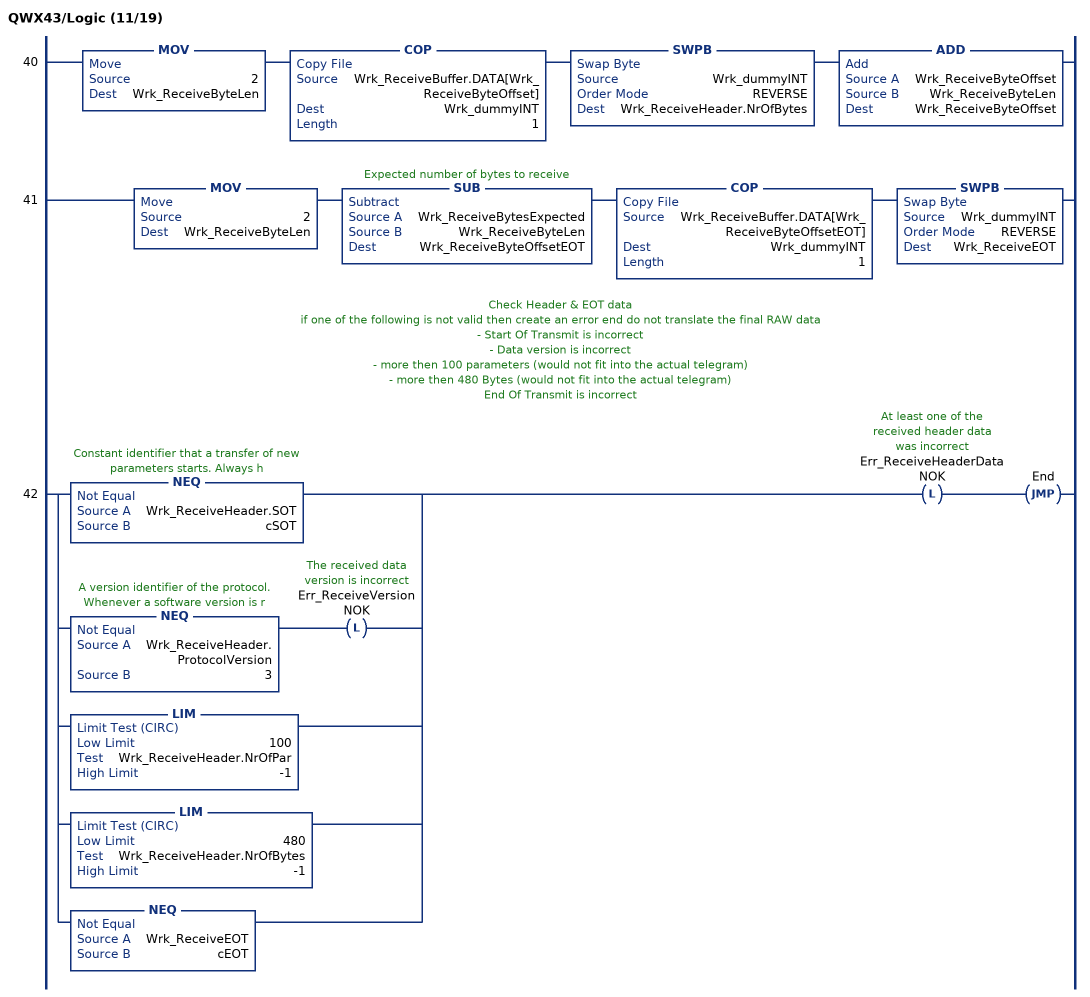
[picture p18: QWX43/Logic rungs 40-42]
   40: MOV(2,Wrk_ReceiveByteLen)COP(Wrk_ReceiveBuffer.DATA[Wrk_ReceiveByteOffset],Wrk_dummyINT,1)SWPB(Wrk_dummyINT,REVERSE,Wrk_ReceiveHeader.NrOfBytes)ADD(Wrk_ReceiveByteOffset,Wrk_ReceiveByteLen,Wrk_ReceiveByteOffset);
   41: MOV(2,Wrk_ReceiveByteLen)SUB(Wrk_ReceiveBytesExpected,Wrk_ReceiveByteLen,Wrk_ReceiveByteOffsetEOT)COP(Wrk_ReceiveBuffer.DATA[Wrk_ReceiveByteOffsetEOT],Wrk_dummyINT,1)SWPB(Wrk_dummyINT,REVERSE,Wrk_ReceiveEOT);
   // Check Header & EOT data
   // if one of the following is not valid then create an error end do not translate the final RAW data
   // - Start Of Transmit is incorrect
   // - Data version is incorrect
   // - more then 100 parameters (would not fit into the actual telegram)
   // - more then 480 Bytes (would not fit into the actual telegram)
   // End Of Transmit is incorrect
   42: [NEQ(Wrk_ReceiveHeader.SOT,cSOT) ,NEQ(Wrk_ReceiveHeader.ProtocolVersion,3) OTL(Err_ReceiveVersionNOK) ,LIM(100,Wrk_ReceiveHeader.NrOfPar,-1) ,LIM(480,Wrk_ReceiveHeader.NrOfBytes,-1) ,NEQ(Wrk_ReceiveEOT,cEOT) ]OTL(Err_ReceiveHeaderDataNOK)JMP(End);
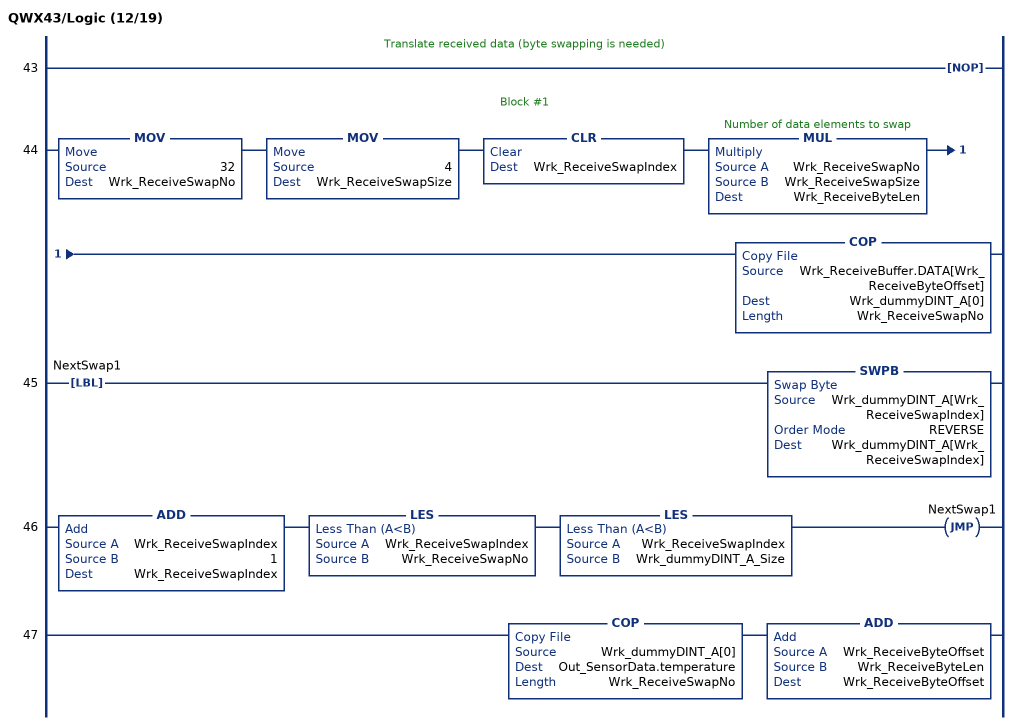
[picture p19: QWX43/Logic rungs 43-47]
   // Translate received data (byte swapping is needed)
   43: NOP();
   // Block #1
   44: MOV(32,Wrk_ReceiveSwapNo)MOV(4,Wrk_ReceiveSwapSize)CLR(Wrk_ReceiveSwapIndex)MUL(Wrk_ReceiveSwapNo,Wrk_ReceiveSwapSize,Wrk_ReceiveByteLen)COP(Wrk_ReceiveBuffer.DATA[Wrk_ReceiveByteOffset],Wrk_dummyDINT_A[0],Wrk_ReceiveSwapNo);
   45: LBL(NextSwap1)SWPB(Wrk_dummyDINT_A[Wrk_ReceiveSwapIndex],REVERSE,Wrk_dummyDINT_A[Wrk_ReceiveSwapIndex]);
   46: ADD(Wrk_ReceiveSwapIndex,1,Wrk_ReceiveSwapIndex)LES(Wrk_ReceiveSwapIndex,Wrk_ReceiveSwapNo)LES(Wrk_ReceiveSwapIndex,Wrk_dummyDINT_A_Size)JMP(NextSwap1);
   47: COP(Wrk_dummyDINT_A[0],Out_SensorData.temperature,Wrk_ReceiveSwapNo)ADD(Wrk_ReceiveByteOffset,Wrk_ReceiveByteLen,Wrk_ReceiveByteOffset);
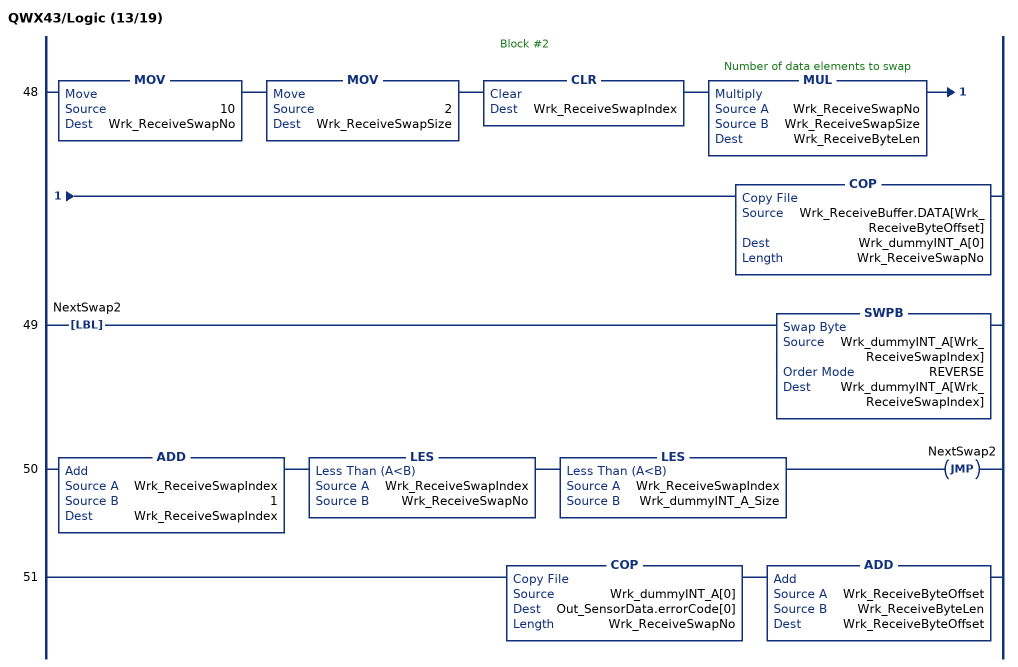
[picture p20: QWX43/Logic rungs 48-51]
   // Block #2
   48: MOV(10,Wrk_ReceiveSwapNo)MOV(2,Wrk_ReceiveSwapSize)CLR(Wrk_ReceiveSwapIndex)MUL(Wrk_ReceiveSwapNo,Wrk_ReceiveSwapSize,Wrk_ReceiveByteLen)COP(Wrk_ReceiveBuffer.DATA[Wrk_ReceiveByteOffset],Wrk_dummyINT_A[0],Wrk_ReceiveSwapNo);
   49: LBL(NextSwap2)SWPB(Wrk_dummyINT_A[Wrk_ReceiveSwapIndex],REVERSE,Wrk_dummyINT_A[Wrk_ReceiveSwapIndex]);
   50: ADD(Wrk_ReceiveSwapIndex,1,Wrk_ReceiveSwapIndex)LES(Wrk_ReceiveSwapIndex,Wrk_ReceiveSwapNo)LES(Wrk_ReceiveSwapIndex,Wrk_dummyINT_A_Size)JMP(NextSwap2);
   51: COP(Wrk_dummyINT_A[0],Out_SensorData.errorCode[0],Wrk_ReceiveSwapNo)ADD(Wrk_ReceiveByteOffset,Wrk_ReceiveByteLen,Wrk_ReceiveByteOffset);
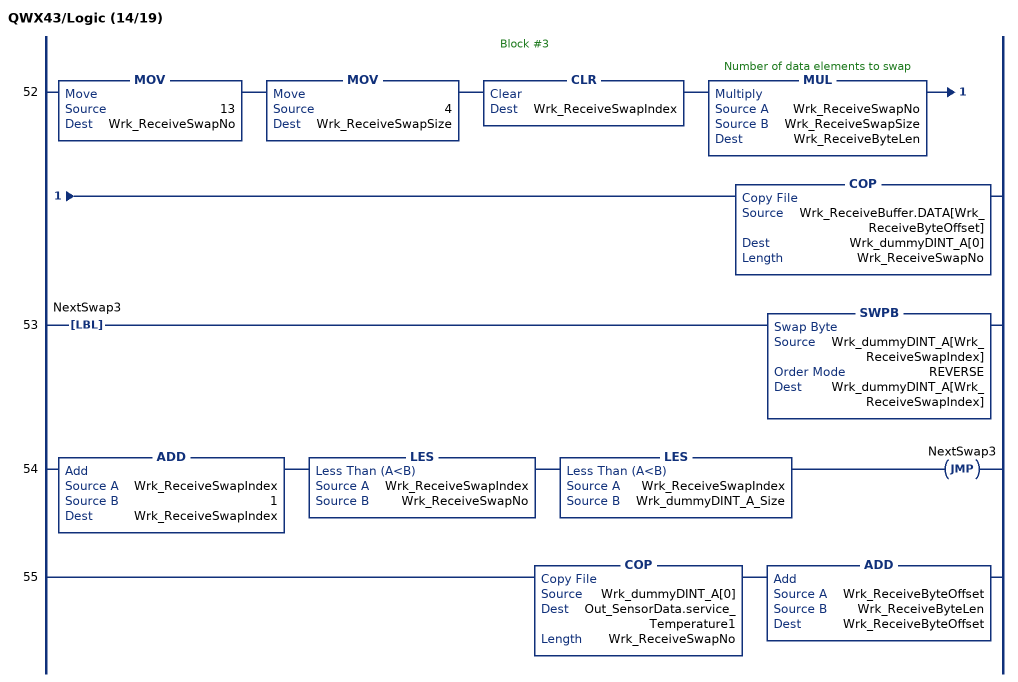
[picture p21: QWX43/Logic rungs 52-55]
   // Block #3
   52: MOV(13,Wrk_ReceiveSwapNo)MOV(4,Wrk_ReceiveSwapSize)CLR(Wrk_ReceiveSwapIndex)MUL(Wrk_ReceiveSwapNo,Wrk_ReceiveSwapSize,Wrk_ReceiveByteLen)COP(Wrk_ReceiveBuffer.DATA[Wrk_ReceiveByteOffset],Wrk_dummyDINT_A[0],Wrk_ReceiveSwapNo);
   53: LBL(NextSwap3)SWPB(Wrk_dummyDINT_A[Wrk_ReceiveSwapIndex],REVERSE,Wrk_dummyDINT_A[Wrk_ReceiveSwapIndex]);
   54: ADD(Wrk_ReceiveSwapIndex,1,Wrk_ReceiveSwapIndex)LES(Wrk_ReceiveSwapIndex,Wrk_ReceiveSwapNo)LES(Wrk_ReceiveSwapIndex,Wrk_dummyDINT_A_Size)JMP(NextSwap3);
   55: COP(Wrk_dummyDINT_A[0],Out_SensorData.service_Temperature1,Wrk_ReceiveSwapNo)ADD(Wrk_ReceiveByteOffset,Wrk_ReceiveByteLen,Wrk_ReceiveByteOffset);
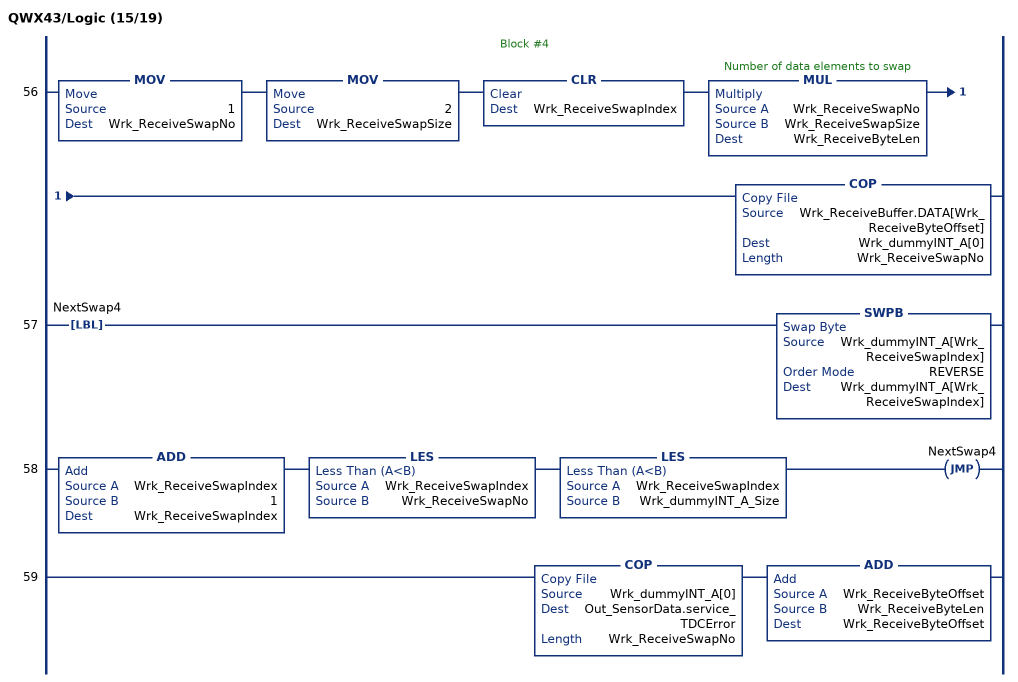
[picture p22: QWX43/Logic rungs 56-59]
   // Block #4
   56: MOV(1,Wrk_ReceiveSwapNo)MOV(2,Wrk_ReceiveSwapSize)CLR(Wrk_ReceiveSwapIndex)MUL(Wrk_ReceiveSwapNo,Wrk_ReceiveSwapSize,Wrk_ReceiveByteLen)COP(Wrk_ReceiveBuffer.DATA[Wrk_ReceiveByteOffset],Wrk_dummyINT_A[0],Wrk_ReceiveSwapNo);
   57: LBL(NextSwap4)SWPB(Wrk_dummyINT_A[Wrk_ReceiveSwapIndex],REVERSE,Wrk_dummyINT_A[Wrk_ReceiveSwapIndex]);
   58: ADD(Wrk_ReceiveSwapIndex,1,Wrk_ReceiveSwapIndex)LES(Wrk_ReceiveSwapIndex,Wrk_ReceiveSwapNo)LES(Wrk_ReceiveSwapIndex,Wrk_dummyINT_A_Size)JMP(NextSwap4);
   59: COP(Wrk_dummyINT_A[0],Out_SensorData.service_TDCError,Wrk_ReceiveSwapNo)ADD(Wrk_ReceiveByteOffset,Wrk_ReceiveByteLen,Wrk_ReceiveByteOffset);
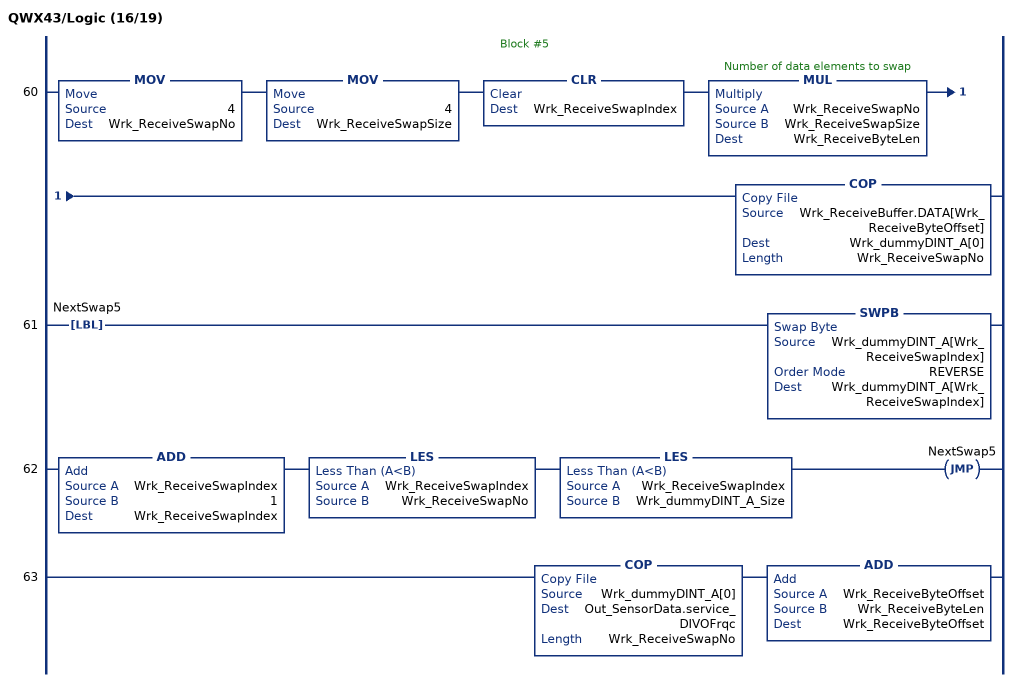
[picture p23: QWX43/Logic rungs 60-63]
   // Block #5
   60: MOV(4,Wrk_ReceiveSwapNo)MOV(4,Wrk_ReceiveSwapSize)CLR(Wrk_ReceiveSwapIndex)MUL(Wrk_ReceiveSwapNo,Wrk_ReceiveSwapSize,Wrk_ReceiveByteLen)COP(Wrk_ReceiveBuffer.DATA[Wrk_ReceiveByteOffset],Wrk_dummyDINT_A[0],Wrk_ReceiveSwapNo);
   61: LBL(NextSwap5)SWPB(Wrk_dummyDINT_A[Wrk_ReceiveSwapIndex],REVERSE,Wrk_dummyDINT_A[Wrk_ReceiveSwapIndex]);
   62: ADD(Wrk_ReceiveSwapIndex,1,Wrk_ReceiveSwapIndex)LES(Wrk_ReceiveSwapIndex,Wrk_ReceiveSwapNo)LES(Wrk_ReceiveSwapIndex,Wrk_dummyDINT_A_Size)JMP(NextSwap5);
   63: COP(Wrk_dummyDINT_A[0],Out_SensorData.service_DIVOFrqc,Wrk_ReceiveSwapNo)ADD(Wrk_ReceiveByteOffset,Wrk_ReceiveByteLen,Wrk_ReceiveByteOffset);
